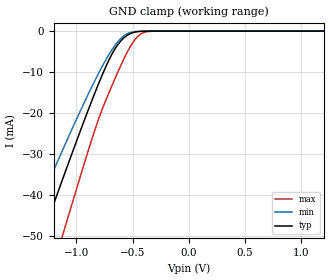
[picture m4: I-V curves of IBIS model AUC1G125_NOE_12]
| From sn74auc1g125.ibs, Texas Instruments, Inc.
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[Model]   AUC1G125_NOE_12
Model_type  Input
Vinl=0.385
Vinh=0.845
| variable   typ   min   max
C_comp   2.21pF   1.84pF   2.74pF
[Temperature Range]   40   100   -40
| Ambient temperature   25   85   -40
[Voltage range]   1.2   1.1   1.3
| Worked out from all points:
|   GND clamp passes 1 mA (typ) near -0.55 V on its own axis
[GND Clamp]
| AUC1G125_NOE_12
|   Voltage   I(typ)   I(min)   I(max)
-3.6V     -230.2mA   -193.8mA   -275.4mA
-1.44V    -60.52mA   -49.07mA   -79.02mA
-1.275V   -47.77mA   -38.55mA   -63.84mA
-1.12V    -35.95mA   -28.87mA   -49.59mA
-1.085V   -33.31mA   -26.72mA   -46.38mA
-820mV    -14.04mA   -11.24mA   -22.86mA
-690mV    -5.96mA    -4.844mA   -13.74mA
-575mV    -1.609mA   -1.103mA   -6.664mA
-495mV    -364.8uA   -190.1uA   -2.692mA
-435mV    -83.65uA   -40.81uA   -873uA
-295mV    -1.276uA   -867.6nA   -9.761uA
1.2V      133.3pA    224.2pA    123.7pA
